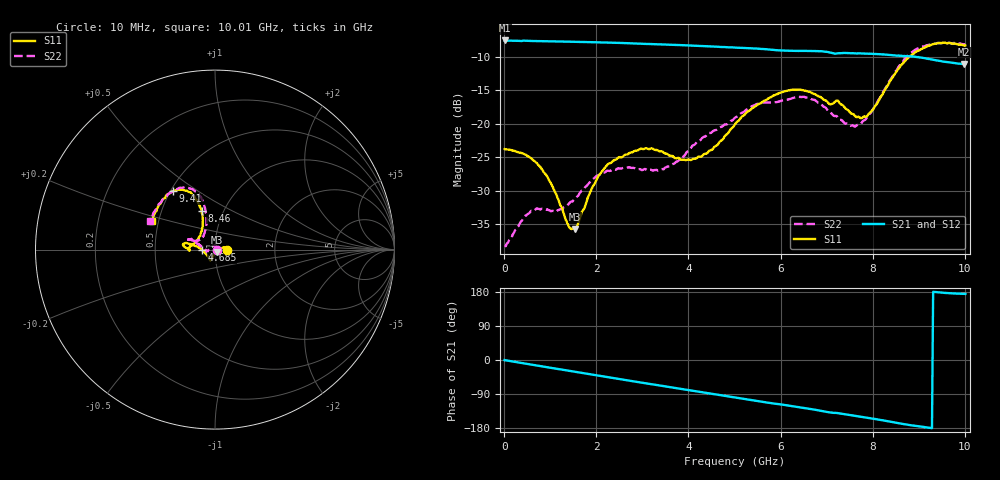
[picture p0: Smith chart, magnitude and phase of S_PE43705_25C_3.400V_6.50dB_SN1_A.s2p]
! Device ID: PE43705
! Serial: 1
! Insertion: A
! Impedance: 50 ohm
! Temp: 25C
! VDD: 3.400V
! Attenuation Step: 6.50dB
#  Hz  S  RI  R  50
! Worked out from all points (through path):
!   401 points, 10 MHz to 10.01 GHz, reference 50 ohm
!   highest |S21| = -7.52 dB at 10 MHz (marker M1); lowest = -11.1 dB at 9.985 GHz (marker M2)
!   group delay of S21, straight-line fit = 53 ps
!   lowest |S11| = -35.8 dB at 1.535 GHz (marker M3), VSWR 1.03, Z = 50.9 - j1.39 ohm
!   |S11| at or under -10 dB: start of sweep to 8.788 GHz
!   |S22| runs from -38.3 to -7.9 dB; largest |S21 - S12| = 0.0041
!   S11 on the Smith chart (normalised r, x): 10 MHz: 1.14, -0.00; 4.685 GHz: 0.86, -0.00; 8.46 GHz: 0.79, +0.36; 9.41 GHz: 0.51, +0.40; 10.01 GHz: 0.46, +0.17
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1e7  0.0647 -0.000162  0.4207 -0.00205  0.4211 -0.00194  0.0122 0.000291
4.6e8  0.0579 0.0109  0.4122 -0.0693  0.4123 -0.0685  0.00941 0.0183
7.6e8  0.047 0.012  0.4007 -0.1114  0.4007 -0.1112  0.00143 0.023
1.385e9  0.0162 -0.00707  0.3638 -0.1938  0.364 -0.1936  -0.021 0.0131
1.535e9  0.00891 -0.0137  0.3522 -0.2118  0.3524 -0.2117  -0.0263 0.00867
1.685e9  0.00159 -0.0219  0.3399 -0.2293  0.3399 -0.2292  -0.0315 0.00314
2.26e9  -0.016 -0.0475  0.2844 -0.289  0.2845 -0.2888  -0.0427 -0.0127
2.935e9  -0.0255 -0.0591  0.2064 -0.3409  0.2071 -0.3409  -0.0443 -0.0118
3.36e9  -0.0272 -0.0564  0.1537 -0.3622  0.1542 -0.3617  -0.0439 -0.00952
4.085e9  -0.0459 -0.0292  0.06 -0.3801  0.0606 -0.38  -0.0679 0.0095
4.685e9  -0.0738 -0.00102  -0.0181 -0.3756  -0.0173 -0.376  -0.0907 0.0269
5.01e9  -0.0977 0.0158  -0.0577 -0.3677  -0.0571 -0.3678  -0.1048 0.037
5.96e9  -0.165 0.0368  -0.1587 -0.3177  -0.1579 -0.3178  -0.1356 0.0564
6.685e9  -0.169 0.014  -0.2255 -0.2685  -0.2254 -0.2684  -0.1419 0.0548
7.635e9  -0.1028 0.046  -0.285 -0.179  -0.2846 -0.1801  -0.068 0.0681
7.91e9  -0.0802 0.0873  -0.2984 -0.1514  -0.2982 -0.153  -0.0566 0.1016
8.36e9  -0.0698 0.1922  -0.3124 -0.0997  -0.312 -0.1008  -0.0506 0.2023
8.46e9  -0.0748 0.2173  -0.3135 -0.0865  -0.3134 -0.0881  -0.0552 0.23
8.885e9  -0.1284 0.3084  -0.3166 -0.0387  -0.3142 -0.04  -0.1167 0.3303
9.41e9  -0.2345 0.3259  -0.2975 0.00695  -0.2965 0.00648  -0.2267 0.3333
9.985e9  -0.3452 0.1684  -0.2787 0.0272  -0.2794 0.0271  -0.3535 0.1723
1.001e10  -0.3525 0.1592  -0.2798 0.0276  -0.2808 0.0274  -0.3611 0.1605
